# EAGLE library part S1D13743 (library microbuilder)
Epson S1D13743 Mobile Graphics Engine with 464K Internal SRAM
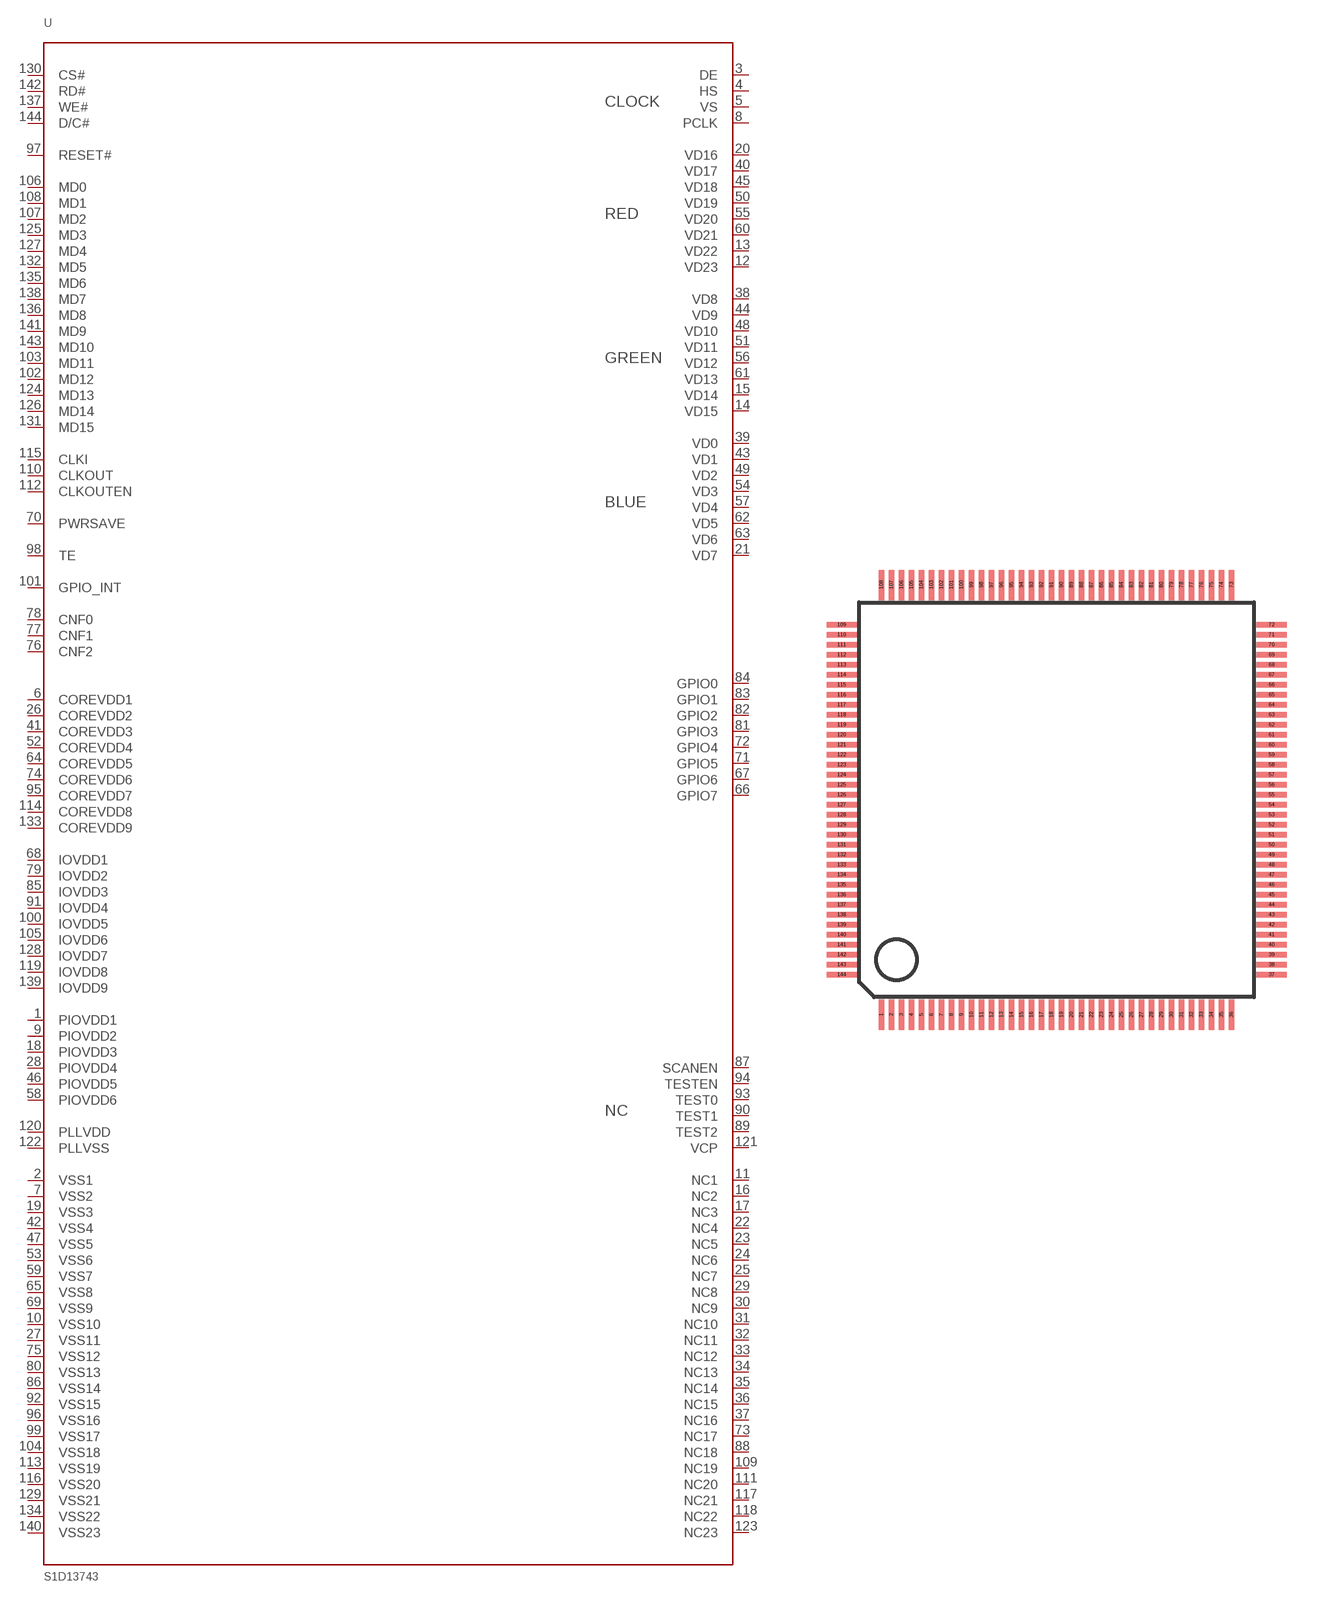
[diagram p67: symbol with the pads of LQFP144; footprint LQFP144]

Designator prefix U

## S1D13743  [LQFP144]
1  PIOVDD1
2  VSS1
3  DE
4  HS
5  VS
6  COREVDD1
7  VSS2
8  PCLK
9  PIOVDD2
10  VSS10
11  NC1
12  VD23
13  VD22
14  VD15
15  VD14
16  NC2
17  NC3
18  PIOVDD3
19  VSS3
20  VD16
21  VD7
22  NC4
23  NC5
24  NC6
25  NC7
26  COREVDD2
27  VSS11
28  PIOVDD4
29  NC8
30  NC9
31  NC10
32  NC11
33  NC12
34  NC13
35  NC14
36  NC15
37  NC16
38  VD8
39  VD0
40  VD17
41  COREVDD3
42  VSS4
43  VD1
44  VD9
45  VD18
46  PIOVDD5
47  VSS5
48  VD10
49  VD2
50  VD19
51  VD11
52  COREVDD4
53  VSS6
54  VD3
55  VD20
56  VD12
57  VD4
58  PIOVDD6
59  VSS7
60  VD21
61  VD13
62  VD5
63  VD6
64  COREVDD5
65  VSS8
66  GPIO7
67  GPIO6
68  IOVDD1
69  VSS9
70  PWRSAVE
71  GPIO5
72  GPIO4
73  NC17
74  COREVDD6
75  VSS12
76  CNF2
77  CNF1
78  CNF0
79  IOVDD2
80  VSS13
81  GPIO3
82  GPIO2
83  GPIO1
84  GPIO0
85  IOVDD3
86  VSS14
87  SCANEN
88  NC18
89  TEST2
90  TEST1
91  IOVDD4
92  VSS15
93  TEST0
94  TESTEN
95  COREVDD7
96  VSS16
97  RESET#
98  TE
99  VSS17
100  IOVDD5
101  GPIO_INT
102  MD12
103  MD11
104  VSS18
105  IOVDD6
106  MD0
107  MD2
108  MD1
109  NC19
110  CLKOUT
111  NC20
112  CLKOUTEN
113  VSS19
114  COREVDD8
115  CLKI
116  VSS20
117  NC21
118  NC22
119  IOVDD8
120  PLLVDD
121  VCP
122  PLLVSS
123  NC23
124  MD13
125  MD3
126  MD14
127  MD4
128  IOVDD7
129  VSS21
130  CS#
131  MD15
132  MD5
133  COREVDD9
134  VSS22
135  MD6
136  MD8
137  WE#
138  MD7
139  IOVDD9
140  VSS23
141  MD9
142  RD#
143  MD10
144  D/C#

## Footprint LQFP144 (pad centres in mm)
Quad Flat Pack
smd 0.27 x 1.5: 1 -8.75,-10.75; 2 -8.25,-10.75; 3 -7.75,-10.75; 4 -7.25,-10.75; 5 -6.75,-10.75; 6 -6.25,-10.75; 7 -5.75,-10.75; 8 -5.25,-10.75; 9 -4.75,-10.75; 10 -4.25,-10.75; 11 -3.75,-10.75; 12 -3.25,-10.75; 13 -2.75,-10.75; 14 -2.25,-10.75; 15 -1.75,-10.75; 16 -1.25,-10.75; 17 -0.75,-10.75; 18 -0.25,-10.75; 19 0.25,-10.75; 20 0.75,-10.75; 21 1.25,-10.75; 22 1.75,-10.75; 23 2.25,-10.75; 24 2.75,-10.75; 25 3.25,-10.75; 26 3.75,-10.75; 27 4.25,-10.75; 28 4.75,-10.75; 29 5.25,-10.75; 30 5.75,-10.75; 31 6.25,-10.75; 32 6.75,-10.75; 33 7.25,-10.75; 34 7.75,-10.75; 35 8.25,-10.75; 36 8.75,-10.75; 73 8.75,10.75; 74 8.25,10.75; 75 7.75,10.75; 76 7.25,10.75; 77 6.75,10.75; 78 6.25,10.75; 79 5.75,10.75; 80 5.25,10.75; 81 4.75,10.75; 82 4.25,10.75; 83 3.75,10.75; 84 3.25,10.75; 85 2.75,10.75; 86 2.25,10.75; 87 1.75,10.75; 88 1.25,10.75; 89 0.75,10.75; 90 0.25,10.75; 91 -0.25,10.75; 92 -0.75,10.75; 93 -1.25,10.75; 94 -1.75,10.75; 95 -2.25,10.75; 96 -2.75,10.75; 97 -3.25,10.75; 98 -3.75,10.75; 99 -4.25,10.75; 100 -4.75,10.75; 101 -5.25,10.75; 102 -5.75,10.75; 103 -6.25,10.75; 104 -6.75,10.75; 105 -7.25,10.75; 106 -7.75,10.75; 107 -8.25,10.75; 108 -8.75,10.75
smd 1.5 x 0.27: 37 10.75,-8.75; 38 10.75,-8.25; 39 10.75,-7.75; 40 10.75,-7.25; 41 10.75,-6.75; 42 10.75,-6.25; 43 10.75,-5.75; 44 10.75,-5.25; 45 10.75,-4.75; 46 10.75,-4.25; 47 10.75,-3.75; 48 10.75,-3.25; 49 10.75,-2.75; 50 10.75,-2.25; 51 10.75,-1.75; 52 10.75,-1.25; 53 10.75,-0.75; 54 10.75,-0.25; 55 10.75,0.25; 56 10.75,0.75; 57 10.75,1.25; 58 10.75,1.75; 59 10.75,2.25; 60 10.75,2.75; 61 10.75,3.25; 62 10.75,3.75; 63 10.75,4.25; 64 10.75,4.75; 65 10.75,5.25; 66 10.75,5.75; 67 10.75,6.25; 68 10.75,6.75; 69 10.75,7.25; 70 10.75,7.75; 71 10.75,8.25; 72 10.75,8.75; 109 -10.75,8.75; 110 -10.75,8.25; 111 -10.75,7.75; 112 -10.75,7.25; 113 -10.75,6.75; 114 -10.75,6.25; 115 -10.75,5.75; 116 -10.75,5.25; 117 -10.75,4.75; 118 -10.75,4.25; 119 -10.75,3.75; 120 -10.75,3.25; 121 -10.75,2.75; 122 -10.75,2.25; 123 -10.75,1.75; 124 -10.75,1.25; 125 -10.75,0.75; 126 -10.75,0.25; 127 -10.75,-0.25; 128 -10.75,-0.75; 129 -10.75,-1.25; 130 -10.75,-1.75; 131 -10.75,-2.25; 132 -10.75,-2.75; 133 -10.75,-3.25; 134 -10.75,-3.75; 135 -10.75,-4.25; 136 -10.75,-4.75; 137 -10.75,-5.25; 138 -10.75,-5.75; 139 -10.75,-6.25; 140 -10.75,-6.75; 141 -10.75,-7.25; 142 -10.75,-7.75; 143 -10.75,-8.25; 144 -10.75,-8.75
